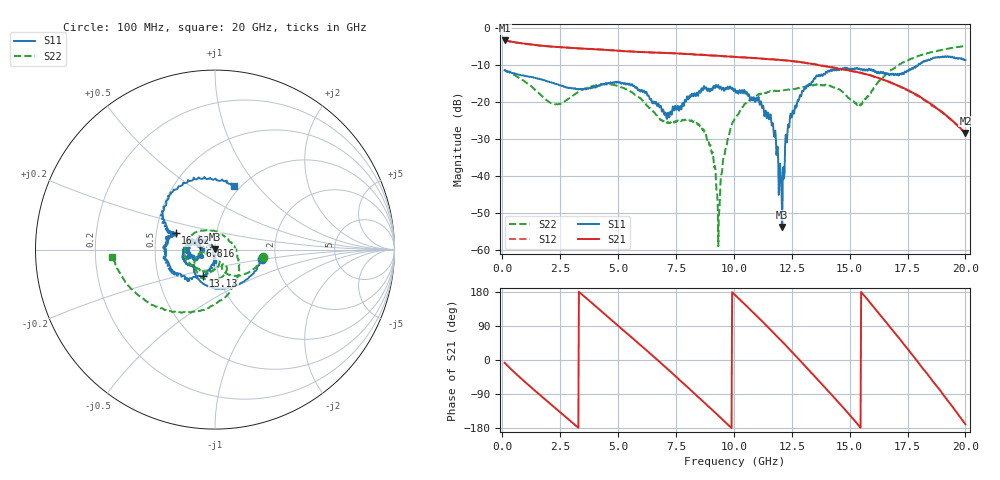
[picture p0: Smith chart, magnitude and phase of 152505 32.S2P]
!  2-Port S-parameters saved by WinCal
! VAR MeasName=S-Parameters (CALIBRATED_DATA) read from VNA (N5230C)
! VAR MeasDate=4/10/2015 9:31:33 AM
! VAR NAME=152505 32
! VAR FILENAME=152505 32.S2P
! VAR DATE=4/10/2015 9:31:33 AM
! VAR PHYS_PORTS=1,2
# Hz S DB R 50
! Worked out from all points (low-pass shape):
!   801 points, 100 MHz to 20 GHz, reference 50 ohm
!   highest |S21| = -3.36 dB at 100 MHz (marker M1); lowest = -28.4 dB at 20 GHz (marker M2)
!   |S21| within 3 dB of the highest: start of sweep to 5.597 GHz
!   lowest |S11| = -53.8 dB at 12.09 GHz (marker M3), VSWR 1.00, Z = 49.9 + j0.15 ohm
!   |S11| at or under -10 dB: start of sweep to 17.96 GHz
!   |S22| runs from -59.1 to -4.8 dB; largest |S21 - S12| = 0.0067
!   S11 on the Smith chart (normalised r, x): 100 MHz: 1.70, -0.20; 6.816 GHz: 0.84, +0.04; 13.13 GHz: 0.84, -0.25; 16.62 GHz: 0.63, +0.12; 20 GHz: 0.94, +0.76
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1e8  -11.40 -11.6  -3.36 -7.5  -3.38 -7.5  -11.31 -9.1
1.617375e9  -13.78 -105.7  -4.74 -91.9  -4.72 -91.7  -17.87 -68.4
3.43325e9  -16.49 -143.5  -5.56 173.3  -5.56 173.4  -16.78 -67.0
4.9755e9  -14.55 -167.0  -6.11 91.7  -6.11 91.4  -15.64 -124.7
6.741625e9  -20.38 164.5  -6.68 -2.2  -6.67 -2.4  -24.23 -166.5
6.81625e9  -21.27 166.2  -6.69 -6.1  -6.68 -6.3  -24.84 -164.1
8.60725e9  -16.31 -165.2  -7.25 -105.8  -7.21 -106.1  -26.74 -173.0
9.079875e9  -16.72 -178.2  -7.46 -132.6  -7.41 -132.5  -33.57 172.4
9.328625e9  -15.45 -175.8  -7.52 -146.8  -7.53 -147.3  -59.05 -81.7
9.627125e9  -16.21 172.8  -7.65 -164.0  -7.63 -164.1  -33.14 -46.1
1.005e10  -16.54 169.6  -7.81 171.6  -7.82 171.3  -24.36 -59.3
1.156738e10  -23.36 125.2  -8.46 80.9  -8.42 81.0  -17.09 -118.0
1.208975e10  -53.83 132.4  -8.73 48.3  -8.66 48.3  -16.98 -132.2
1.2438e10  -23.33 -92.6  -8.87 25.8  -8.94 25.7  -16.62 -136.9
1.31345e10  -15.96 -114.4  -9.46 -19.5  -9.47 -19.4  -15.93 -152.7
1.338325e10  -14.51 -123.1  -9.74 -35.9  -9.68 -35.6  -15.46 -160.3
1.427875e10  -11.18 -154.9  -10.72 -95.5  -10.63 -96.1  -15.97 159.9
1.5423e10  -10.93 176.3  -12.06 -175.2  -12.04 -176.3  -21.16 46.9
1.6617e10  -12.52 157.6  -14.32 96.8  -14.38 96.1  -12.24 -69.6
1.669162e10  -12.70 159.5  -14.52 90.9  -14.64 89.9  -11.78 -72.9
1.8408e10  -8.55 140.3  -20.15 -41.0  -20.31 -42.3  -6.74 -137.2
2e10  -8.69 73.4  -28.42 -169.5  -28.48 -168.7  -4.84 -175.8
